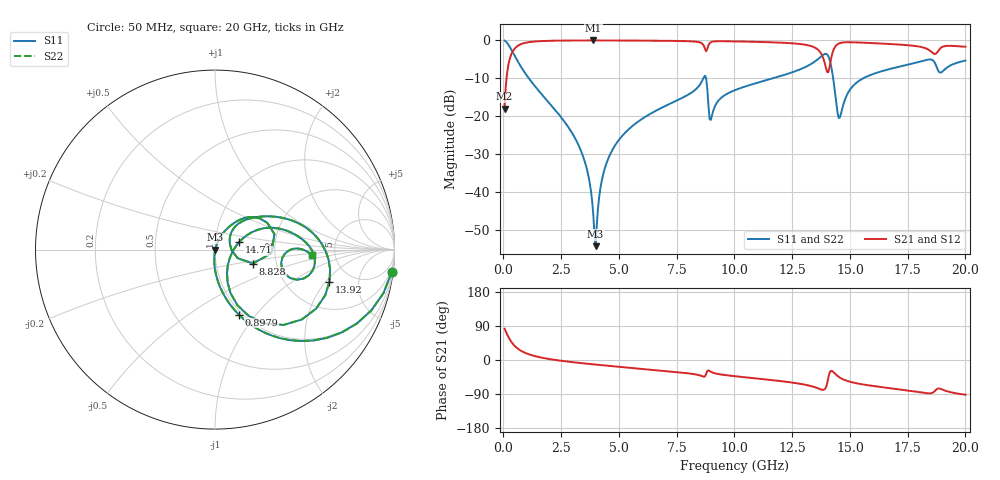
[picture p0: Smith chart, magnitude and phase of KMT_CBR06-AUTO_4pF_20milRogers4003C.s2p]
! Data measured by Modelithics Inc. support@modelithics.com 813-866-6335
! KEMET CBR06-AUTO 4pF, Pad Width= 0.851mm, Pad Length= 0.64mm, Pad Gap= 0.62mm, 20mil Rogers 4003C substrate Data, January 2022
# hz S ma R 50
! 2 Port Network Data from SP1.SP block
! freq  magS11  angS11  magS21  angS21  magS12  angS12  magS22  angS22
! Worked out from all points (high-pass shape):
!   401 points, 50 MHz to 20 GHz, reference 50 ohm
!   highest |S21| = -0.02 dB at 3.89 GHz (marker M1); lowest = -18.0 dB at 50 MHz (marker M2)
!   |S21| within 3 dB of the highest: 392 MHz to 13.7 GHz (13.31 GHz wide, 189 % of centre); 14.26 GHz to 18.53 GHz (4.27 GHz wide, 26 % of centre)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
!   lowest |S11| = -54.3 dB at 3.99 GHz (marker M3), VSWR 1.00, Z = 50.2 + j0.0149 ohm
!   |S11| at or under -10 dB: 1.097 GHz to 8.655 GHz (7.558 GHz wide, 155 % of centre); 8.776 GHz to 11.67 GHz (2.89 GHz wide, 28.3 % of centre); 14.27 GHz to 15.58 GHz (1.305 GHz wide, 8.74 % of centre)
!   |S22| runs from -54.3 to -0.1 dB; largest |S21 - S12| = 0
!   S11 on the Smith chart (normalised r, x): 50 MHz: 1, -15; 897.9 MHz: 0.96, -0.82; 8.828 GHz: 1.51, -0.25; 13.92 GHz: 3.44, -2.19; 14.71 GHz: 1.31, +0.11; 20 GHz: 3.33, -0.30
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5e7  0.992 -7.4  0.1256 82.6  0.1256 82.6  0.992 -7.4
3.4925e8  0.7462 -42.7  0.6648 47.2  0.6648 47.2  0.7462 -42.7
8.97875e8  0.3855 -69.9  0.9216 20.0  0.9216 20.0  0.3855 -69.9
3.391625e9  0.03276 -95.4  0.9976 -8.4  0.9976 -8.4  0.03276 -95.4
3.690875e9  0.01555 -93.7  0.998 -10.3  0.998 -10.3  0.01555 -93.7
3.890375e9  0.005008 -80.2  0.998 -11.5  0.998 -11.5  0.005008 -80.2
3.990125e9  0.001925 4.4  0.998 -12.1  0.998 -12.1  0.001925 4.4
4.289375e9  0.01569 69.1  0.9978 -13.9  0.9978 -13.9  0.01569 69.1
4.73825e9  0.03684 70.4  0.9971 -16.4  0.9971 -16.4  0.03684 70.4
6.73325e9  0.1238 61.3  0.9894 -27.4  0.9894 -27.4  0.1238 61.3
8.678375e9  0.3272 27.2  0.8457 -44.1  0.8457 -44.1  0.3272 27.2
8.828e9  0.2252 -20.1  0.7763 -28.4  0.7763 -28.4  0.2252 -20.1
9.0275e9  0.1019 36.5  0.9588 -32.6  0.9588 -32.6  0.1019 36.5
1.0025e10  0.2206 45.8  0.9698 -42.8  0.9698 -42.8  0.2206 45.8
1.336662e10  0.498 16.3  0.8323 -69.6  0.8323 -69.6  0.498 16.3
1.391525e10  0.6623 -15.6  0.4957 -77.0  0.4957 -77.0  0.6623 -15.6
1.416462e10  0.4955 -56.1  0.5322 -29.2  0.5322 -29.2  0.4955 -56.1
1.451375e10  0.09498 -30.6  0.907 -44.5  0.907 -44.5  0.09498 -30.6
1.471325e10  0.1412 17.3  0.9392 -51.3  0.9392 -51.3  0.1412 17.3
1.670825e10  0.4178 14.3  0.8973 -74.2  0.8973 -74.2  0.4178 14.3
1.870325e10  0.4872 -20.2  0.6623 -80.2  0.6623 -80.2  0.4872 -20.2
2e10  0.5411 -3.4  0.8241 -91.7  0.8241 -91.7  0.5411 -3.4
